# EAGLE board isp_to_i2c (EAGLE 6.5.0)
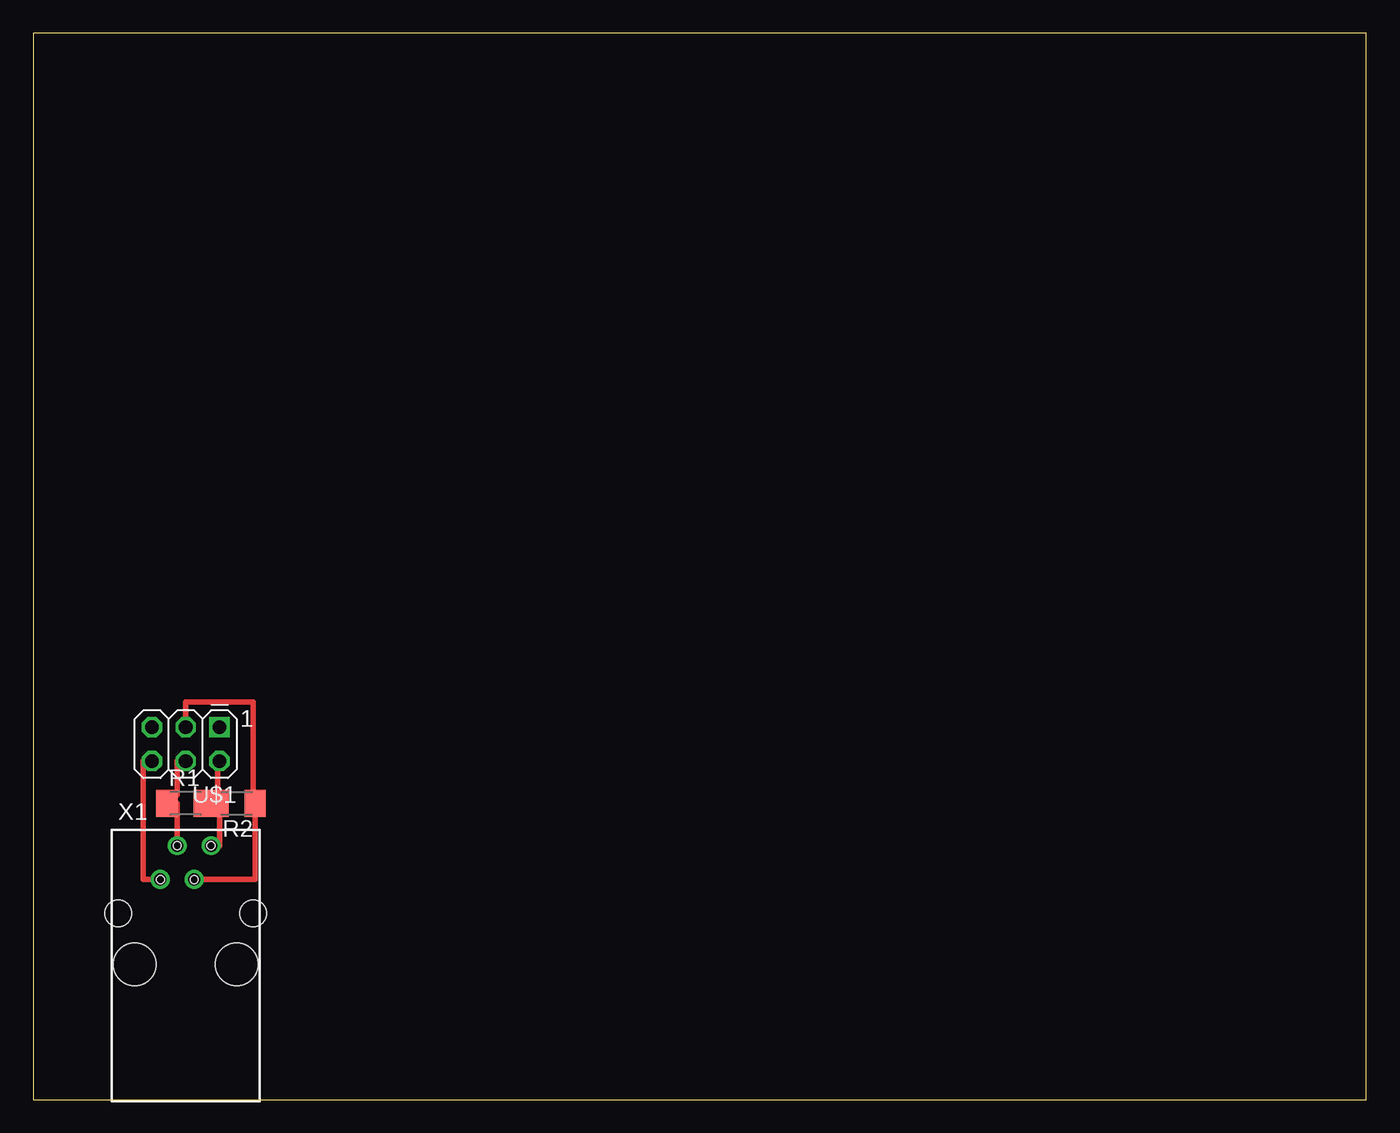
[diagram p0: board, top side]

Size 100 x 80 mm. Coordinates in mm from the lower left corner, seen from the top.
Outline: 0,0 100,0 100,80 0,80 0,0
Copper layers (1*16): Top 0.035mm / dielectric 1.5mm / Bottom 0.035mm
Design rules "default": minimum track width 10mil, minimum drill 24mil, track to track 8mil, track to pad 8mil, pad to pad 8mil, via to via 8mil, smd to smd 8mil, copper to edge 40mil, drill to drill 8mil, minimum pad ring 10mil, minimum via ring 8mil, stop-mask expansion 4mil, vias tented up to drill 0mil, thermal gap 10mil
Holes 0.6 mm at 9.53,16.51 12.06,16.51 13.34,19.05 10.79,19.05
Holes 2 mm at 16.51,13.97 6.35,13.97

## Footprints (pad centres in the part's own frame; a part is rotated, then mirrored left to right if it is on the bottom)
M1206 = smd 1.6 x 2: 1 -1.4,0; 2 1.4,0
2X03 = drill 1.016 square: 1 -2.54,-1.27 | drill 1.016 octagon: 2 -2.54,1.27; 3 0,-1.27; 4 0,1.27; 5 2.54,-1.27; 6 2.54,1.27
14867 = drill 0.9 pad 1.422: 1 -1.905,6.35; 2 -0.635,8.89; 3 0.635,6.35; 4 1.905,8.89 | hole 3.2: -3.81,0; 3.81,0

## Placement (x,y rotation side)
R1  10k  [M1206]  11.43,22.23 0 top
R2  10k  [M1206]  15.24,22.23 180 top
U$1  AVRISP  [2X03]  11.43,26.67 180 top
X1  14867  [14867]  11.43,10.16 0 top

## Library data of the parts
R1 R2 = resistor
U$1 = fab
X1 = con-4ucon; OC_FARNELL: unknown; OC_NEWARK: unknown

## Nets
GND: U$1.6 X1.1
SCL: R1.1 U$1.4 X1.2
SDA: R2.1 U$1.3 X1.3
VCC: R1.2 R2.2 U$1.2 X1.4

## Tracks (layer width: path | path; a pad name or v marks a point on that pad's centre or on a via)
GND
  Top 0.406: U$1.6 8.26,25.4 8.26,16.51 X1.1
SCL
  Top 0.406: U$1.4 10.79,25.4 10.79,22.86 10.03,22.86 R1.1 10.79,22.23 X1.2
SDA
  Top 0.406: X1.3 16.64,16.51 R2.1 16.51,22.23 16.51,29.84 11.43,29.84 U$1.3
VCC
  Top 0.406: U$1.2 13.84,25.4 R2.2 R1.2 13.97,22.23 13.97,19.05 X1.4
